(* Logix 5000 AddOnInstructionDefinition export SPEL_Above; software revision 30.01; part 4 of 9 *)

ADD_ON_INSTRUCTION SPEL_Jog   (* revision 1.0, vendor SEIKO EPSON CORP. *)
// Jogs the robot.
VAR_INPUT
   Start : BOOL; {required}
   MaxTime : DINT := 30000; {access None, visible}
END_VAR
VAR_OUTPUT
   InCycle : BOOL; {access Read Only, visible}
   Done : BOOL; {access Read Only, visible}
   Error : BOOL; {access Read Only, visible}
END_VAR
VAR_INPUT
   JogMode : INT; {required}
   Axis : INT; {required}
   Distance : REAL; {required}
END_VAR
VAR_IN_OUT
   ExtInputs : AB:ETHERNET_MODULE_INT_128Bytes:I:0; {required}
   ExtOutputs : AB:ETHERNET_MODULE_INT_128Bytes:O:0; {required}
END_VAR
VAR_OUTPUT
   ErrCode1 : INT; {access Read Only, visible}
   ErrCode2 : INT; {access Read Only, visible}
END_VAR
VAR
   ExecJog : SPEL_ExecCmd := (MaxTime := 3000); {access None}
   Distance_INTS : INT[2]; {access None}
   StartInit : BOOL; {access None}
   OneShotStart : BOOL; {access None}
   Distancex1000 : DINT; {access None}
   ExecTimeout : DINT; {access None}
END_VAR

ROUTINE Logic   (* ladder *)
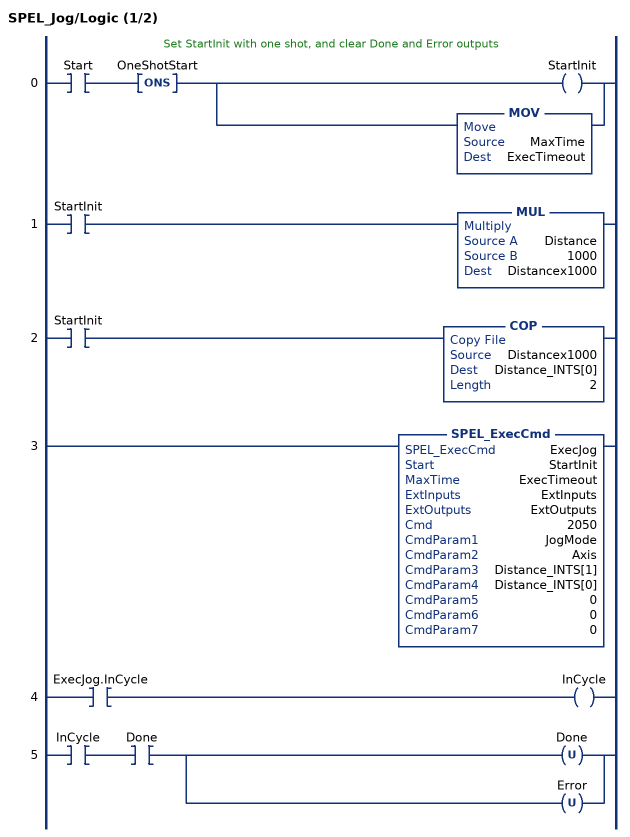
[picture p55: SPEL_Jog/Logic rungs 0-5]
   // Set StartInit with one shot, and clear Done and Error outputs
   0: XIC(Start)ONS(OneShotStart)[OTE(StartInit) ,MOV(MaxTime,ExecTimeout) ];
   1: XIC(StartInit)MUL(Distance,1000,Distancex1000);
   2: XIC(StartInit)COP(Distancex1000,Distance_INTS[0],2);
   3: SPEL_ExecCmd(ExecJog,StartInit,ExecTimeout,ExtInputs,ExtOutputs,2050,JogMode,Axis,Distance_INTS[1],Distance_INTS[0],0,0,0);
   4: XIC(ExecJog.InCycle)OTE(InCycle);
   5: XIC(InCycle)XIC(Done)[OTU(Done) ,OTU(Error) ];
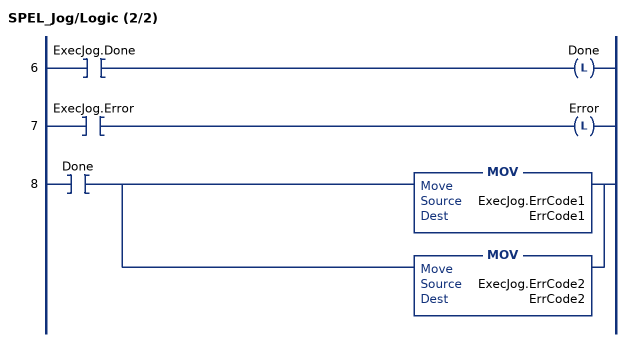
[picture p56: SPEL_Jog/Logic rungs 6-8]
   6: XIC(ExecJog.Done)OTL(Done);
   7: XIC(ExecJog.Error)OTL(Error);
   8: XIC(Done)[MOV(ExecJog.ErrCode1,ErrCode1) ,MOV(ExecJog.ErrCode2,ErrCode2) ];
END_ROUTINE
END_ADD_ON_INSTRUCTION

ADD_ON_INSTRUCTION SPEL_Jump   (* revision 1.0, vendor SEIKO EPSON CORP. *)
// Moves the arm in gate trajectory using PTP motion.
VAR_OUTPUT
   InCycle : BOOL; {access Read Only, visible}
   Done : BOOL; {access Read Only, visible}
   Error : BOOL; {access Read Only, visible}
END_VAR
VAR_INPUT
   Start : BOOL; {required}
   MaxTime : DINT := 30000; {access None, visible}
   TargetType : INT; {access None, visible}
   ArchNum : INT := 7; {access None, visible}
   Point : INT; {required}
   PalletNum : INT; {access None, visible}
   PalletPosOrCol : INT; {access None, visible}
   PalletRow : INT; {access None, visible}
END_VAR
VAR_IN_OUT
   ExtInputs : AB:ETHERNET_MODULE_INT_128Bytes:I:0; {required}
   ExtOutputs : AB:ETHERNET_MODULE_INT_128Bytes:O:0; {required}
END_VAR
VAR_OUTPUT
   ErrCode1 : INT; {access Read Only, visible}
   ErrCode2 : INT; {access Read Only, visible}
END_VAR
VAR
   ExecJump : SPEL_ExecCmd := (MaxTime := 3000, CmdParam1 := 112); {access None}
   StartInit : BOOL; {access None}
   CmdParam1 : INT; {access None}
   PointOrPalletNum : INT; {access None}
   BSL_Control : CONTROL; {access None}
   BSL_SourceBit : BOOL; {access None}
   Local_Arch : DINT; {access None}
   OneShotStart : BOOL; {access None}
   ExecTimeout : DINT; {access None}
   OneShotCP : BOOL; {access None}
   Local_CP : DINT; {access None}
   LocalCP : DINT; {access None}
   ArchError : BOOL; {access None}
   StartExec : BOOL; {access None}
   ExecuteCmd : BOOL; {access None}
   TargetTypeError : BOOL; {access None}
   OneShotArch : BOOL; {access None}
   OneShotTargetType : BOOL; {access None}
END_VAR

ROUTINE Logic   (* ladder *)
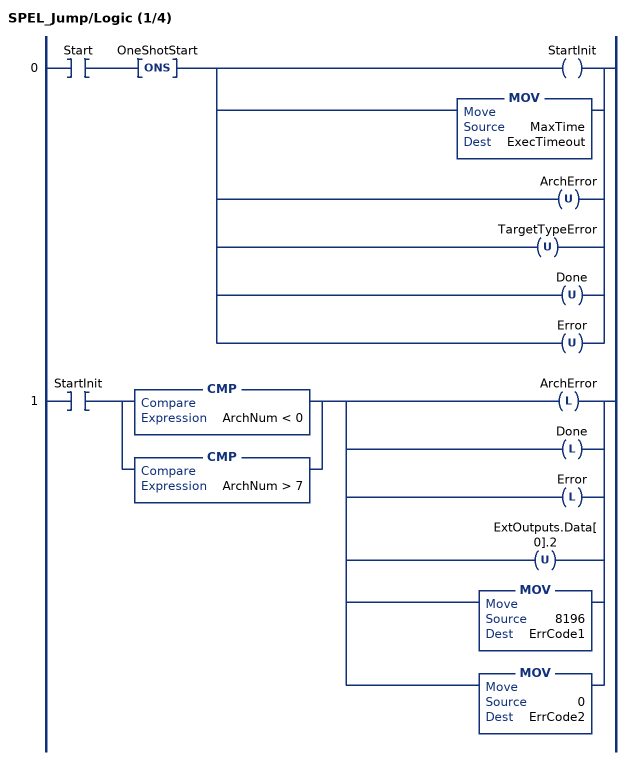
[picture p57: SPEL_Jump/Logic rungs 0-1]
   0: XIC(Start)ONS(OneShotStart)[OTE(StartInit) ,MOV(MaxTime,ExecTimeout) ,OTU(ArchError) ,OTU(TargetTypeError) ,OTU(Done) ,OTU(Error) ];
   1: XIC(StartInit)[CMP(ArchNum < 0) ,CMP(ArchNum > 7) ][OTL(ArchError) ,OTL(Done) ,OTL(Error) ,OTU(ExtOutputs.Data[0].2) ,MOV(8196,ErrCode1) ,MOV(0,ErrCode2) ];
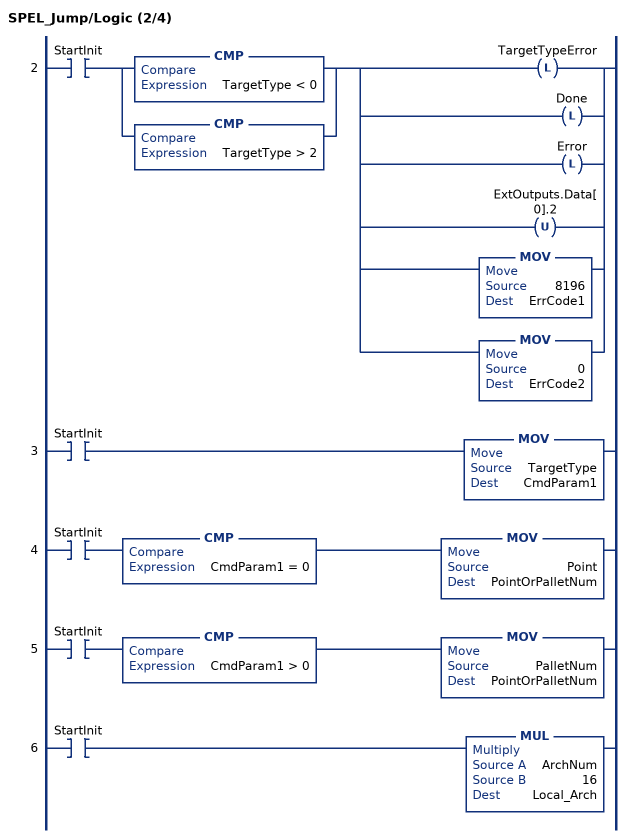
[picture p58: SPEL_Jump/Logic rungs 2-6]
   2: XIC(StartInit)[CMP(TargetType < 0) ,CMP(TargetType > 2) ][OTL(TargetTypeError) ,OTL(Done) ,OTL(Error) ,OTU(ExtOutputs.Data[0].2) ,MOV(8196,ErrCode1) ,MOV(0,ErrCode2) ];
   3: XIC(StartInit)MOV(TargetType,CmdParam1);
   4: XIC(StartInit)CMP(CmdParam1 = 0)MOV(Point,PointOrPalletNum);
   5: XIC(StartInit)CMP(CmdParam1 > 0)MOV(PalletNum,PointOrPalletNum);
   6: XIC(StartInit)MUL(ArchNum,16,Local_Arch);
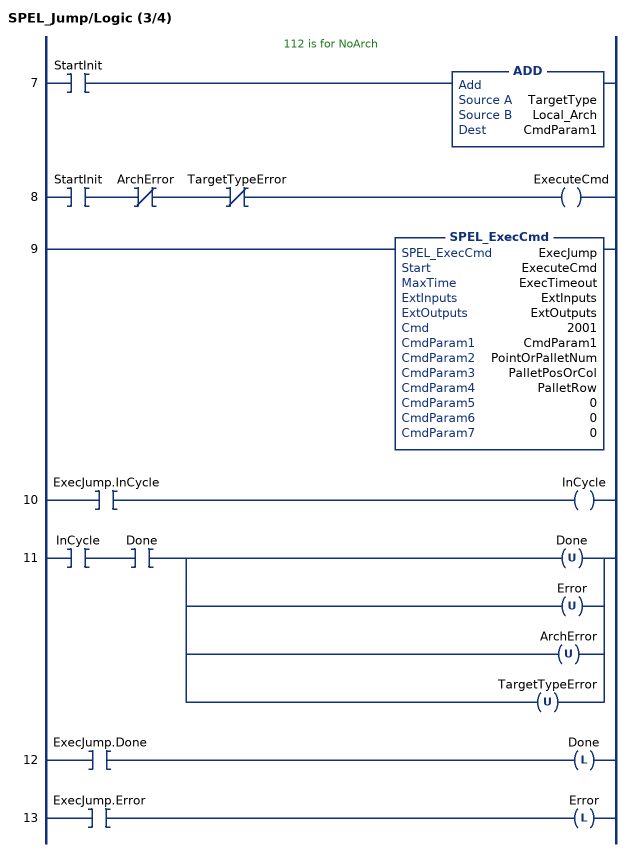
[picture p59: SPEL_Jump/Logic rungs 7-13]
   // 112 is for NoArch
   7: XIC(StartInit)ADD(TargetType,Local_Arch,CmdParam1);
   8: XIC(StartInit)XIO(ArchError)XIO(TargetTypeError)OTE(ExecuteCmd);
   9: SPEL_ExecCmd(ExecJump,ExecuteCmd,ExecTimeout,ExtInputs,ExtOutputs,2001,CmdParam1,PointOrPalletNum,PalletPosOrCol,PalletRow,0,0,0);
   10: XIC(ExecJump.InCycle)OTE(InCycle);
   11: XIC(InCycle)XIC(Done)[OTU(Done) ,OTU(Error) ,OTU(ArchError) ,OTU(TargetTypeError) ];
   12: XIC(ExecJump.Done)OTL(Done);
   13: XIC(ExecJump.Error)OTL(Error);
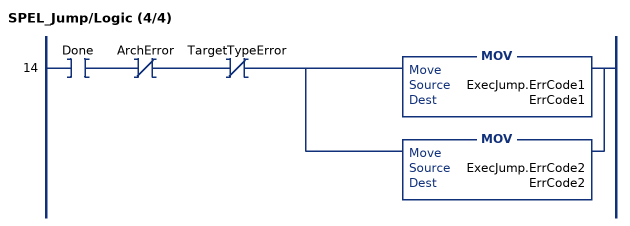
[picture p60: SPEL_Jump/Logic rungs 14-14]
   14: XIC(Done)XIO(ArchError)XIO(TargetTypeError)[MOV(ExecJump.ErrCode1,ErrCode1) ,MOV(ExecJump.ErrCode2,ErrCode2) ];
END_ROUTINE
END_ADD_ON_INSTRUCTION

ADD_ON_INSTRUCTION SPEL_Jump3   (* revision 1.0, vendor SEIKO EPSON CORP. *)
// Moves the arm with 3D gate motion
// This is a combination of two CP motion and one PTP motion.
VAR_OUTPUT
   InCycle : BOOL; {access Read Only, visible}
   Done : BOOL; {access Read Only, visible}
   Error : BOOL; {access Read Only, visible}
END_VAR
VAR_INPUT
   Start : BOOL; {required}
   MaxTime : DINT := 30000; {access None, visible}
   ArchNum : DINT := 7; {access None, visible}
   DepartPoint : INT; {required}
   ApproPoint : INT; {required}
   DestPoint : INT; {required}
END_VAR
VAR_IN_OUT
   ExtInputs : AB:ETHERNET_MODULE_INT_128Bytes:I:0; {required}
   ExtOutputs : AB:ETHERNET_MODULE_INT_128Bytes:O:0; {required}
END_VAR
VAR_OUTPUT
   ErrCode1 : INT; {access Read Only, visible}
   ErrCode2 : INT; {access Read Only, visible}
END_VAR
VAR
   ExecJump3 : SPEL_ExecCmd := (MaxTime := 3000, CmdParam1 := 112); {access None}
   OneShotStart : BOOL; {access None}
   StartInit : BOOL; {access None}
   ExecTimeout : DINT; {access None}
   Local_Arch : DINT; {access None}
   CmdParam1 : DINT; {access None}
   ArchError : BOOL; {access None}
   StartExec : BOOL; {access None}
   ExecuteCmd : BOOL; {access None}
   OneShotArch : BOOL; {access None}
END_VAR

ROUTINE Logic   (* ladder *)
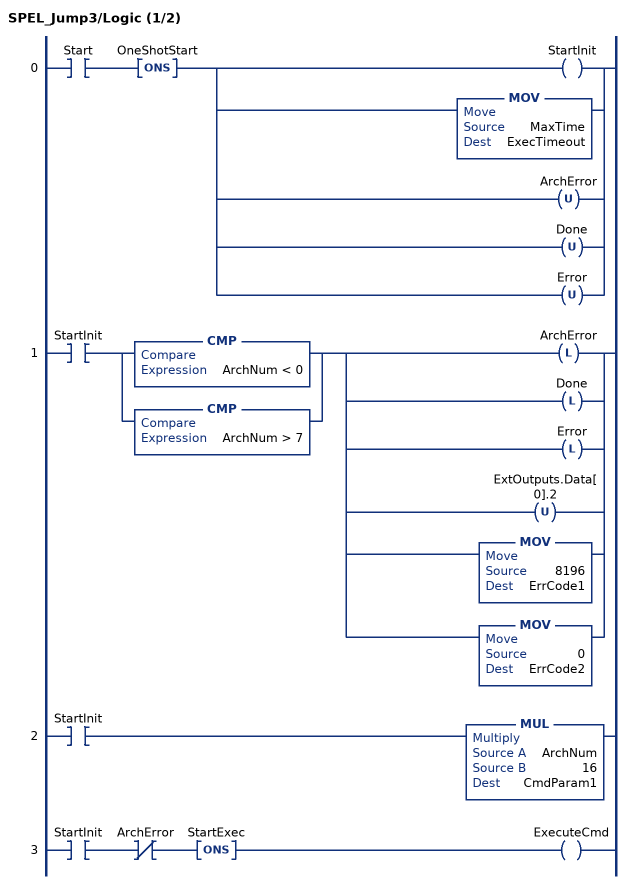
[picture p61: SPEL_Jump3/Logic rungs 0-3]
   0: XIC(Start)ONS(OneShotStart)[OTE(StartInit) ,MOV(MaxTime,ExecTimeout) ,OTU(ArchError) ,OTU(Done) ,OTU(Error) ];
   1: XIC(StartInit)[CMP(ArchNum < 0) ,CMP(ArchNum > 7) ][OTL(ArchError) ,OTL(Done) ,OTL(Error) ,OTU(ExtOutputs.Data[0].2) ,MOV(8196,ErrCode1) ,MOV(0,ErrCode2) ];
   2: XIC(StartInit)MUL(ArchNum,16,CmdParam1);
   3: XIC(StartInit)XIO(ArchError)ONS(StartExec)OTE(ExecuteCmd);
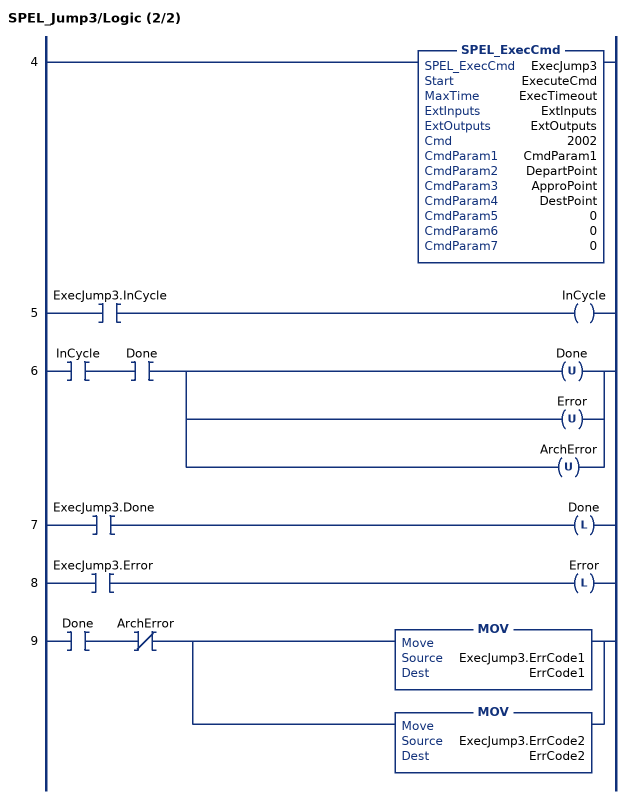
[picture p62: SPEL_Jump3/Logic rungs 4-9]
   4: SPEL_ExecCmd(ExecJump3,ExecuteCmd,ExecTimeout,ExtInputs,ExtOutputs,2002,CmdParam1,DepartPoint,ApproPoint,DestPoint,0,0,0);
   5: XIC(ExecJump3.InCycle)OTE(InCycle);
   6: XIC(InCycle)XIC(Done)[OTU(Done) ,OTU(Error) ,OTU(ArchError) ];
   7: XIC(ExecJump3.Done)OTL(Done);
   8: XIC(ExecJump3.Error)OTL(Error);
   9: XIC(Done)XIO(ArchError)[MOV(ExecJump3.ErrCode1,ErrCode1) ,MOV(ExecJump3.ErrCode2,ErrCode2) ];
END_ROUTINE
END_ADD_ON_INSTRUCTION

ADD_ON_INSTRUCTION SPEL_Jump3CP   (* revision 1.0, vendor SEIKO EPSON CORP. *)
// Moves the manipulator in 3D gate trajectory, using three CP motions.
VAR_OUTPUT
   InCycle : BOOL; {access Read Only, visible}
   Done : BOOL; {access Read Only, visible}
   Error : BOOL; {access Read Only, visible}
END_VAR
VAR_INPUT
   Start : BOOL; {required}
   MaxTime : DINT := 120000; {access None, visible}
   ArchNum : DINT := 7; {access None, visible}
   DepartPoint : INT; {required}
   ApproPoint : INT; {required}
   DestPoint : INT; {required}
END_VAR
VAR_IN_OUT
   ExtInputs : AB:ETHERNET_MODULE_INT_128Bytes:I:0; {required}   // ExtReset Bit
   ExtOutputs : AB:ETHERNET_MODULE_INT_128Bytes:O:0; {required}
END_VAR
VAR_OUTPUT
   ErrCode1 : INT; {access Read Only, visible}
   ErrCode2 : INT; {access Read Only, visible}
END_VAR
VAR
   ExecJump3CP : SPEL_ExecCmd := (MaxTime := 3000, CmdParam1 := 112); {access None}
   OneShotStart : BOOL; {access None}
   StartInit : BOOL; {access None}
   ExecTimeout : DINT; {access None}
   Local_Arch : DINT; {access None}
   CmdParam1 : DINT; {access None}
   StartExec : BOOL; {access None}
   ExecuteCmd : BOOL; {access None}
   ArchError : BOOL; {access None}
   OneShotArch : BOOL; {access None}
END_VAR

ROUTINE Logic   (* ladder *)
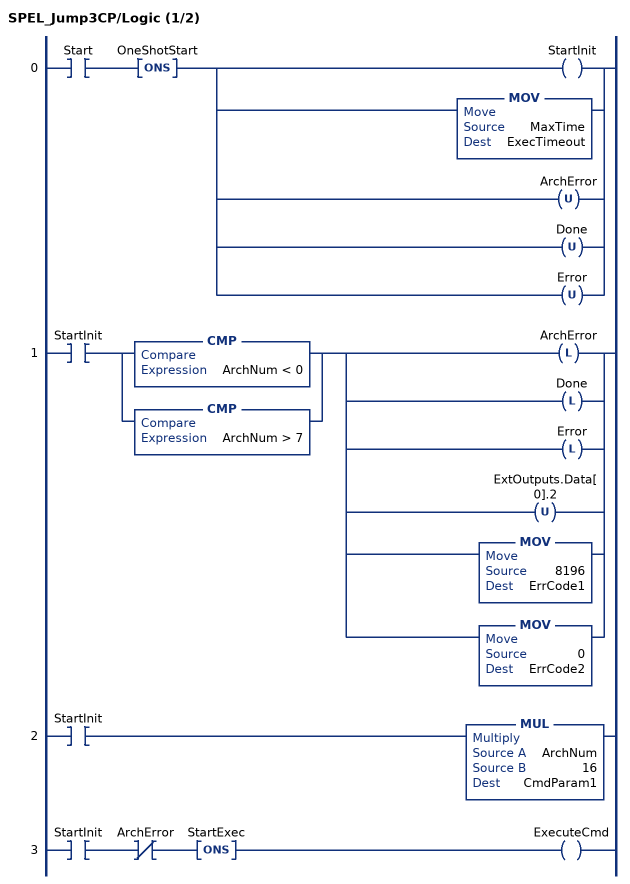
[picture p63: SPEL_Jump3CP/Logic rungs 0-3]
   0: XIC(Start)ONS(OneShotStart)[OTE(StartInit) ,MOV(MaxTime,ExecTimeout) ,OTU(ArchError) ,OTU(Done) ,OTU(Error) ];
   1: XIC(StartInit)[CMP(ArchNum < 0) ,CMP(ArchNum > 7) ][OTL(ArchError) ,OTL(Done) ,OTL(Error) ,OTU(ExtOutputs.Data[0].2) ,MOV(8196,ErrCode1) ,MOV(0,ErrCode2) ];
   2: XIC(StartInit)MUL(ArchNum,16,CmdParam1);
   3: XIC(StartInit)XIO(ArchError)ONS(StartExec)OTE(ExecuteCmd);
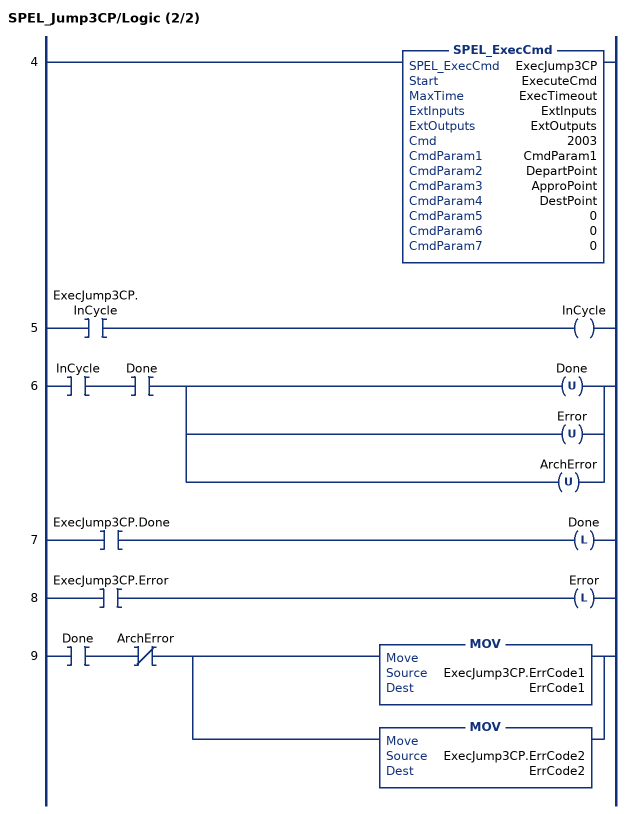
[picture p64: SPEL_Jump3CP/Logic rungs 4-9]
   4: SPEL_ExecCmd(ExecJump3CP,ExecuteCmd,ExecTimeout,ExtInputs,ExtOutputs,2003,CmdParam1,DepartPoint,ApproPoint,DestPoint,0,0,0);
   5: XIC(ExecJump3CP.InCycle)OTE(InCycle);
   6: XIC(InCycle)XIC(Done)[OTU(Done) ,OTU(Error) ,OTU(ArchError) ];
   7: XIC(ExecJump3CP.Done)OTL(Done);
   8: XIC(ExecJump3CP.Error)OTL(Error);
   9: XIC(Done)XIO(ArchError)[MOV(ExecJump3CP.ErrCode1,ErrCode1) ,MOV(ExecJump3CP.ErrCode2,ErrCode2) ];
END_ROUTINE
END_ADD_ON_INSTRUCTION

ADD_ON_INSTRUCTION SPEL_Lefty   (* revision 1.0, vendor SEIKO EPSON CORP. *)
// Sets the hand orientation of the specified point to Lefty.
VAR_OUTPUT
   InCycle : BOOL; {access Read Only, visible}
   Done : BOOL; {access Read Only, visible}
   Error : BOOL; {access Read Only, visible}
END_VAR
VAR_INPUT
   Start : BOOL; {required}
   Point : INT; {required}
END_VAR
VAR_IN_OUT
   ExtInputs : AB:ETHERNET_MODULE_INT_128Bytes:I:0; {required}
   ExtOutputs : AB:ETHERNET_MODULE_INT_128Bytes:O:0; {required}
END_VAR
VAR_OUTPUT
   ErrCode1 : INT; {access Read Only, visible}
   ErrCode2 : INT; {access Read Only, visible}
END_VAR
VAR
   ExecLefty : SPEL_ExecCmd := (MaxTime := 3000); {access None}
   height_INTS : INT[2]; {access None}
   OneShotStart : BOOL; {access None}
   StartCoil : BOOL; {access None}
   ExecTimeout : DINT; {access None}
END_VAR

ROUTINE Logic   (* ladder *)
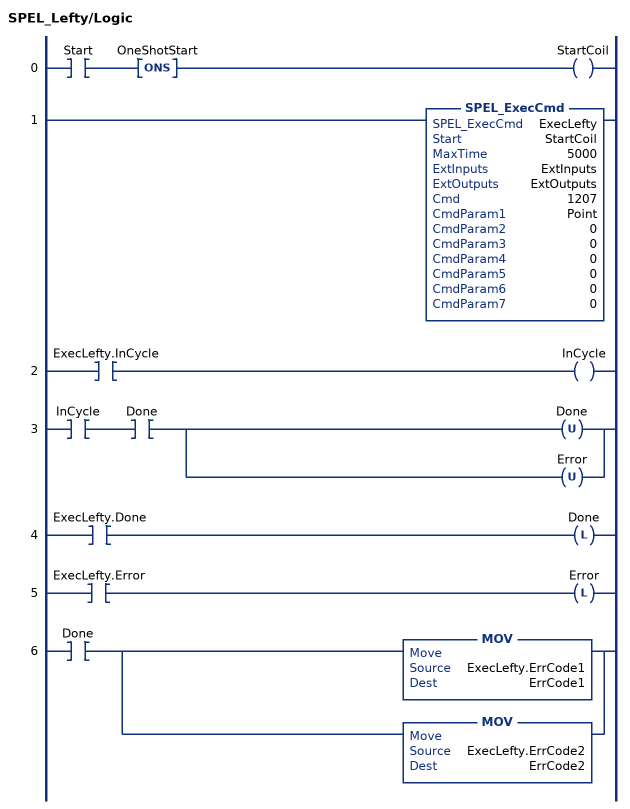
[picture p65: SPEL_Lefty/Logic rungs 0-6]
   0: XIC(Start)ONS(OneShotStart)OTE(StartCoil);
   1: SPEL_ExecCmd(ExecLefty,StartCoil,5000,ExtInputs,ExtOutputs,1207,Point,0,0,0,0,0,0);
   2: XIC(ExecLefty.InCycle)OTE(InCycle);
   3: XIC(InCycle)XIC(Done)[OTU(Done) ,OTU(Error) ];
   4: XIC(ExecLefty.Done)OTL(Done);
   5: XIC(ExecLefty.Error)OTL(Error);
   6: XIC(Done)[MOV(ExecLefty.ErrCode1,ErrCode1) ,MOV(ExecLefty.ErrCode2,ErrCode2) ];
END_ROUTINE
END_ADD_ON_INSTRUCTION

ADD_ON_INSTRUCTION SPEL_LimZ   (* revision 1.0, vendor SEIKO EPSON CORP. *)
// Sets the initial Joint #3 height (Z coordinate value) in Jump command.
VAR_OUTPUT
   InCycle : BOOL; {access Read Only, visible}
   Done : BOOL; {access Read Only, visible}
   Error : BOOL; {access Read Only, visible}
END_VAR
VAR_INPUT
   Start : BOOL; {required}
   Height : REAL; {required}
END_VAR
VAR_IN_OUT
   ExtInputs : AB:ETHERNET_MODULE_INT_128Bytes:I:0; {required}
   ExtOutputs : AB:ETHERNET_MODULE_INT_128Bytes:O:0; {required}
END_VAR
VAR_OUTPUT
   ErrCode1 : INT; {access Read Only, visible}
   ErrCode2 : INT; {access Read Only, visible}
END_VAR
VAR
   ExecLimZ : SPEL_ExecCmd := (MaxTime := 3000); {access None}
   StartInit : BOOL; {access None}
   OneShotStart : BOOL; {access None}
   heightx1000 : DINT; {access None}
   height_INTS : INT[2]; {access None}
   ExecTimeout : DINT; {access None}
END_VAR

ROUTINE Logic   (* ladder *)
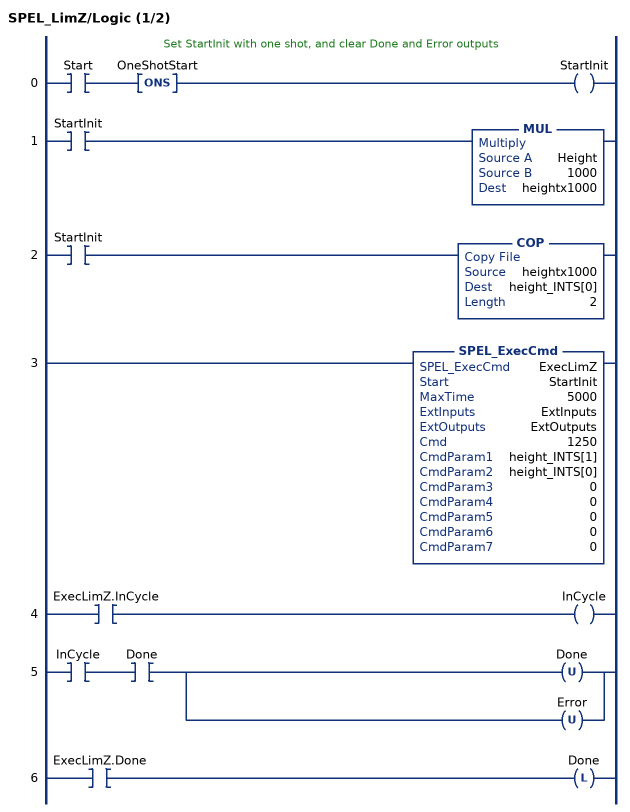
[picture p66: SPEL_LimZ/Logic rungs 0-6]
   // Set StartInit with one shot, and clear Done and Error outputs
   0: XIC(Start)ONS(OneShotStart)OTE(StartInit);
   1: XIC(StartInit)MUL(Height,1000,heightx1000);
   2: XIC(StartInit)COP(heightx1000,height_INTS[0],2);
   3: SPEL_ExecCmd(ExecLimZ,StartInit,5000,ExtInputs,ExtOutputs,1250,height_INTS[1],height_INTS[0],0,0,0,0,0);
   4: XIC(ExecLimZ.InCycle)OTE(InCycle);
   5: XIC(InCycle)XIC(Done)[OTU(Done) ,OTU(Error) ];
   6: XIC(ExecLimZ.Done)OTL(Done);
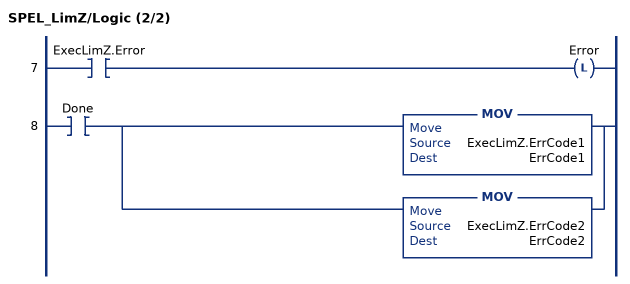
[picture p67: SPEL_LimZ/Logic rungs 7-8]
   7: XIC(ExecLimZ.Error)OTL(Error);
   8: XIC(Done)[MOV(ExecLimZ.ErrCode1,ErrCode1) ,MOV(ExecLimZ.ErrCode2,ErrCode2) ];
END_ROUTINE
END_ADD_ON_INSTRUCTION

ADD_ON_INSTRUCTION SPEL_LocalGet   (* revision 1.0, vendor SEIKO EPSON CORP. *)
// Gets the setting status of the Local coordinate system number.
VAR_INPUT
   Start : BOOL; {required}
END_VAR
VAR_OUTPUT
   InCycle : BOOL; {access Read Only, visible}
   Done : BOOL; {access Read Only, visible}
   Error : BOOL; {access Read Only, visible}
END_VAR
VAR_INPUT
   NumAxes : INT; {required}
   LocalNum : INT; {required}
END_VAR
VAR_OUTPUT
   LocalX : REAL; {visible}
   LocalY : REAL; {visible}
   LocalZ : REAL; {visible}
   LocalU : REAL; {visible}
   LocalV : REAL; {visible}
   LocalW : REAL; {visible}
END_VAR
VAR_IN_OUT
   ExtInputs : AB:ETHERNET_MODULE_INT_128Bytes:I:0; {required}
   ExtOutputs : AB:ETHERNET_MODULE_INT_128Bytes:O:0; {required}
END_VAR
VAR_OUTPUT
   ErrCode1 : INT; {access Read Only, visible}
   ErrCode2 : INT; {access Read Only, visible}
END_VAR
VAR
   Coordinatex1000 : DINT; {access None}
   Coordinate_INTS : INT[2]; {access None}
   ExecLocalGetZ : SPEL_ExecCmd := (MaxTime := 3000); {access None}
   ExecLocalGetY : SPEL_ExecCmd := (MaxTime := 3000); {access None}
   ExecLocalGetX : SPEL_ExecCmd := (MaxTime := 3000); {access None}
   X6 : BOOL; {access None}
   StartInit : BOOL[32]; {access None}
   OneShotStart : BOOL[32]; {access None}
   ExecLocalGetW : SPEL_ExecCmd := (MaxTime := 3000); {access None}
   ExecLocalGetV : SPEL_ExecCmd := (MaxTime := 3000); {access None}
   ExecLocalGetU : SPEL_ExecCmd := (MaxTime := 3000); {access None}
   ExecTimeout : DINT; {access None}
END_VAR

ROUTINE Logic   (* ladder *)
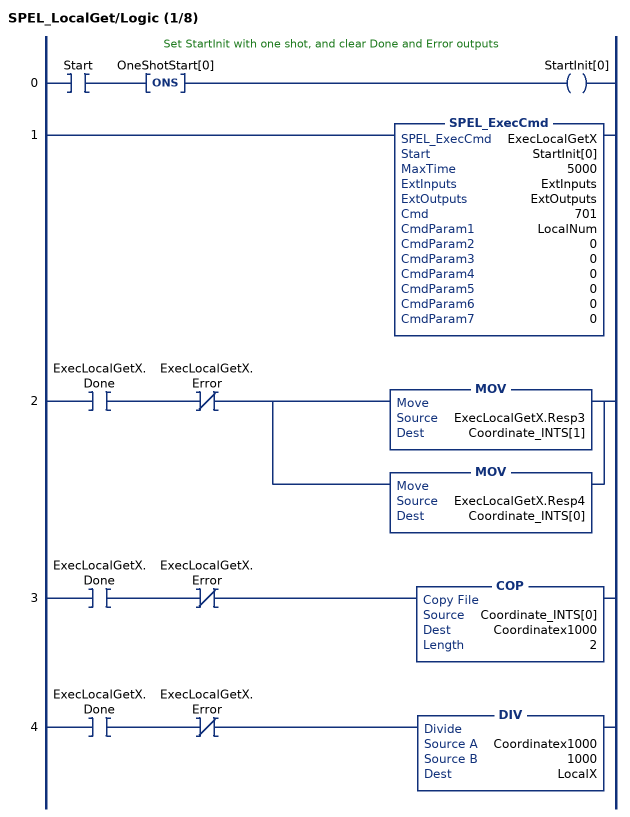
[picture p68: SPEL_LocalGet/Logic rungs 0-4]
   // Set StartInit with one shot, and clear Done and Error outputs
   0: XIC(Start)ONS(OneShotStart[0])OTE(StartInit[0]);
   1: SPEL_ExecCmd(ExecLocalGetX,StartInit[0],5000,ExtInputs,ExtOutputs,701,LocalNum,0,0,0,0,0,0);
   2: XIC(ExecLocalGetX.Done)XIO(ExecLocalGetX.Error)[MOV(ExecLocalGetX.Resp3,Coordinate_INTS[1]) ,MOV(ExecLocalGetX.Resp4,Coordinate_INTS[0]) ];
   3: XIC(ExecLocalGetX.Done)XIO(ExecLocalGetX.Error)COP(Coordinate_INTS[0],Coordinatex1000,2);
   4: XIC(ExecLocalGetX.Done)XIO(ExecLocalGetX.Error)DIV(Coordinatex1000,1000,LocalX);
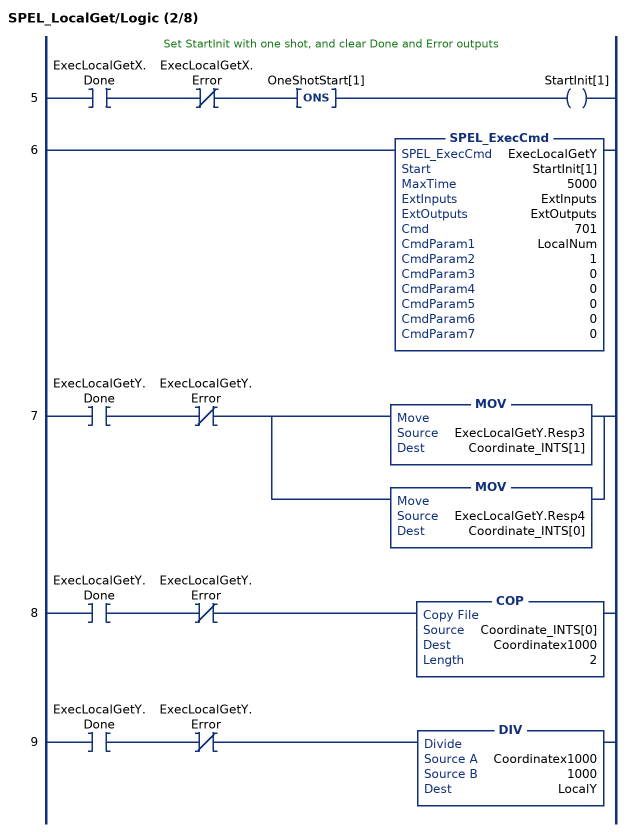
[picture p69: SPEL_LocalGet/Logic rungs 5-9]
   // Set StartInit with one shot, and clear Done and Error outputs
   5: XIC(ExecLocalGetX.Done)XIO(ExecLocalGetX.Error)ONS(OneShotStart[1])OTE(StartInit[1]);
   6: SPEL_ExecCmd(ExecLocalGetY,StartInit[1],5000,ExtInputs,ExtOutputs,701,LocalNum,1,0,0,0,0,0);
   7: XIC(ExecLocalGetY.Done)XIO(ExecLocalGetY.Error)[MOV(ExecLocalGetY.Resp3,Coordinate_INTS[1]) ,MOV(ExecLocalGetY.Resp4,Coordinate_INTS[0]) ];
   8: XIC(ExecLocalGetY.Done)XIO(ExecLocalGetY.Error)COP(Coordinate_INTS[0],Coordinatex1000,2);
   9: XIC(ExecLocalGetY.Done)XIO(ExecLocalGetY.Error)DIV(Coordinatex1000,1000,LocalY);
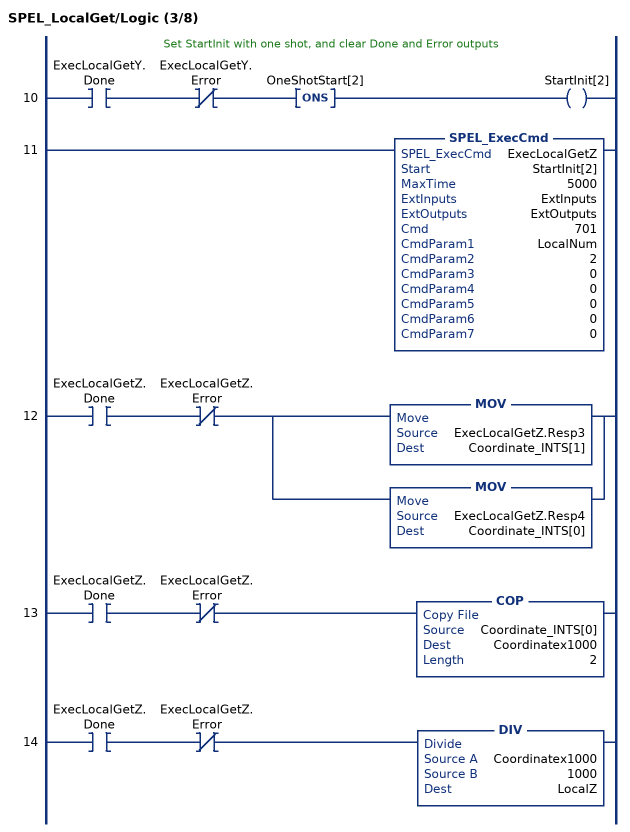
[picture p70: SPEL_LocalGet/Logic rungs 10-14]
   // Set StartInit with one shot, and clear Done and Error outputs
   10: XIC(ExecLocalGetY.Done)XIO(ExecLocalGetY.Error)ONS(OneShotStart[2])OTE(StartInit[2]);
   11: SPEL_ExecCmd(ExecLocalGetZ,StartInit[2],5000,ExtInputs,ExtOutputs,701,LocalNum,2,0,0,0,0,0);
   12: XIC(ExecLocalGetZ.Done)XIO(ExecLocalGetZ.Error)[MOV(ExecLocalGetZ.Resp3,Coordinate_INTS[1]) ,MOV(ExecLocalGetZ.Resp4,Coordinate_INTS[0]) ];
   13: XIC(ExecLocalGetZ.Done)XIO(ExecLocalGetZ.Error)COP(Coordinate_INTS[0],Coordinatex1000,2);
   14: XIC(ExecLocalGetZ.Done)XIO(ExecLocalGetZ.Error)DIV(Coordinatex1000,1000,LocalZ);
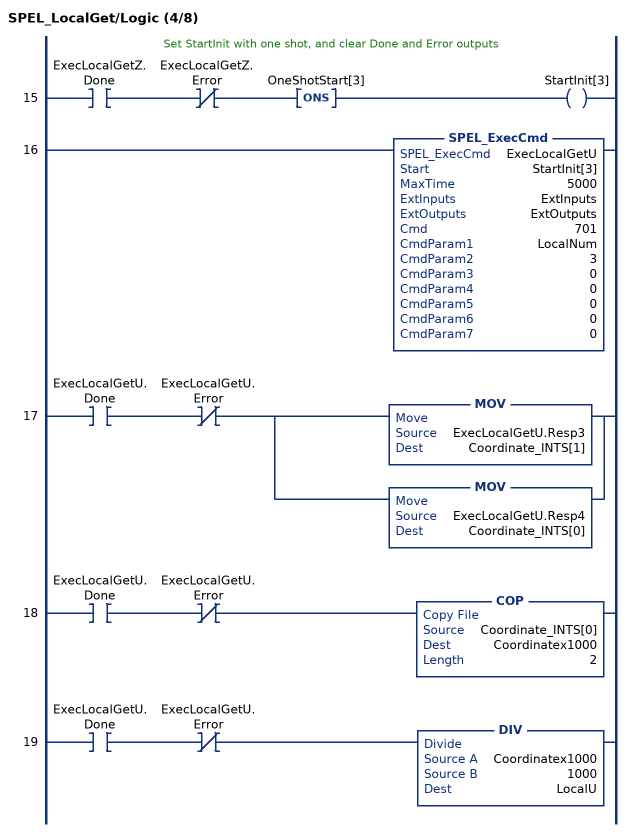
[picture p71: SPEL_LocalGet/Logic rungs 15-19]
   // Set StartInit with one shot, and clear Done and Error outputs
   15: XIC(ExecLocalGetZ.Done)XIO(ExecLocalGetZ.Error)ONS(OneShotStart[3])OTE(StartInit[3]);
   16: SPEL_ExecCmd(ExecLocalGetU,StartInit[3],5000,ExtInputs,ExtOutputs,701,LocalNum,3,0,0,0,0,0);
   17: XIC(ExecLocalGetU.Done)XIO(ExecLocalGetU.Error)[MOV(ExecLocalGetU.Resp3,Coordinate_INTS[1]) ,MOV(ExecLocalGetU.Resp4,Coordinate_INTS[0]) ];
   18: XIC(ExecLocalGetU.Done)XIO(ExecLocalGetU.Error)COP(Coordinate_INTS[0],Coordinatex1000,2);
   19: XIC(ExecLocalGetU.Done)XIO(ExecLocalGetU.Error)DIV(Coordinatex1000,1000,LocalU);
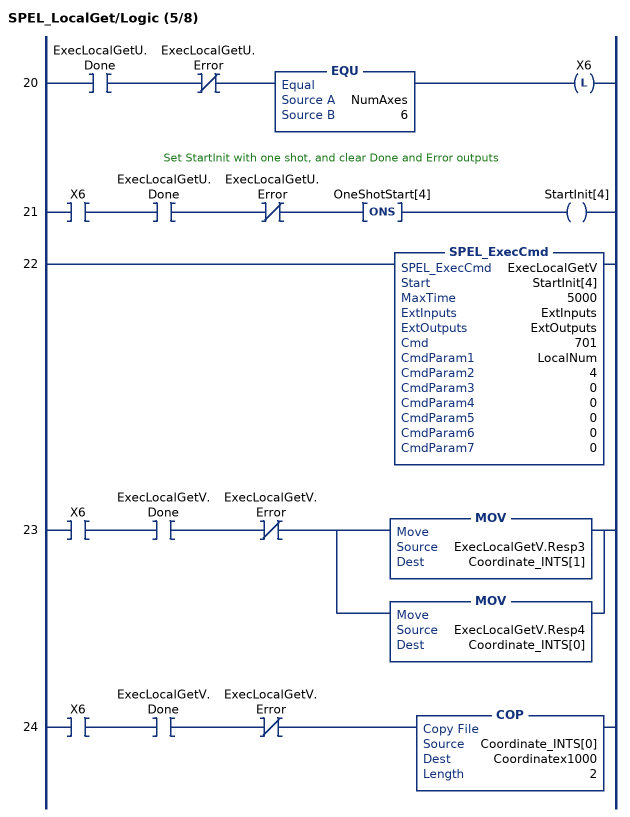
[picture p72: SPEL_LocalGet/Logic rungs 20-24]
   20: XIC(ExecLocalGetU.Done)XIO(ExecLocalGetU.Error)EQU(NumAxes,6)OTL(X6);
   // Set StartInit with one shot, and clear Done and Error outputs
   21: XIC(X6)XIC(ExecLocalGetU.Done)XIO(ExecLocalGetU.Error)ONS(OneShotStart[4])OTE(StartInit[4]);
   22: SPEL_ExecCmd(ExecLocalGetV,StartInit[4],5000,ExtInputs,ExtOutputs,701,LocalNum,4,0,0,0,0,0);
   23: XIC(X6)XIC(ExecLocalGetV.Done)XIO(ExecLocalGetV.Error)[MOV(ExecLocalGetV.Resp3,Coordinate_INTS[1]) ,MOV(ExecLocalGetV.Resp4,Coordinate_INTS[0]) ];
   24: XIC(X6)XIC(ExecLocalGetV.Done)XIO(ExecLocalGetV.Error)COP(Coordinate_INTS[0],Coordinatex1000,2);
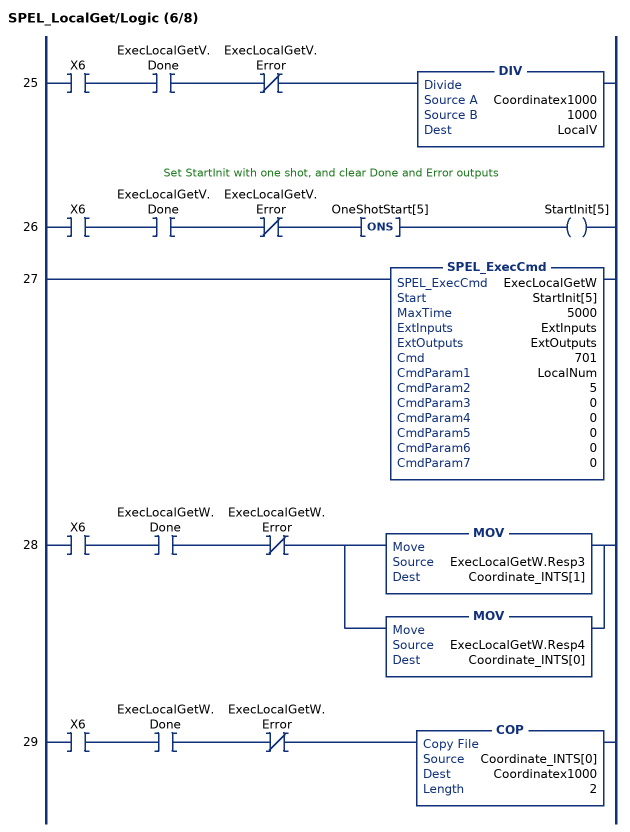
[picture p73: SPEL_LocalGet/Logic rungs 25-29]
   25: XIC(X6)XIC(ExecLocalGetV.Done)XIO(ExecLocalGetV.Error)DIV(Coordinatex1000,1000,LocalV);
   // Set StartInit with one shot, and clear Done and Error outputs
   26: XIC(X6)XIC(ExecLocalGetV.Done)XIO(ExecLocalGetV.Error)ONS(OneShotStart[5])OTE(StartInit[5]);
   27: SPEL_ExecCmd(ExecLocalGetW,StartInit[5],5000,ExtInputs,ExtOutputs,701,LocalNum,5,0,0,0,0,0);
   28: XIC(X6)XIC(ExecLocalGetW.Done)XIO(ExecLocalGetW.Error)[MOV(ExecLocalGetW.Resp3,Coordinate_INTS[1]) ,MOV(ExecLocalGetW.Resp4,Coordinate_INTS[0]) ];
   29: XIC(X6)XIC(ExecLocalGetW.Done)XIO(ExecLocalGetW.Error)COP(Coordinate_INTS[0],Coordinatex1000,2);
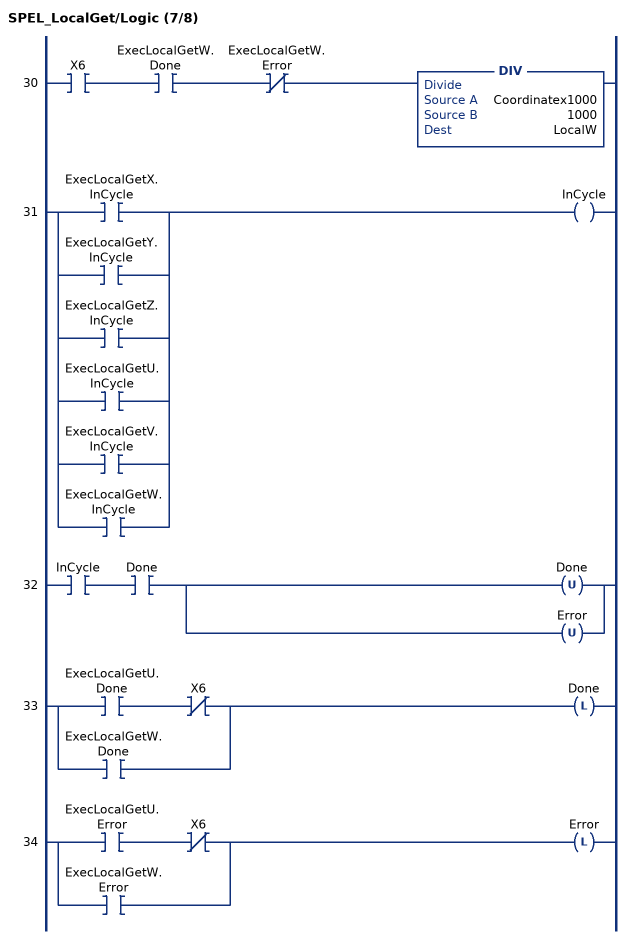
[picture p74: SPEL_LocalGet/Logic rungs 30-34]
   30: XIC(X6)XIC(ExecLocalGetW.Done)XIO(ExecLocalGetW.Error)DIV(Coordinatex1000,1000,LocalW);
   31: [XIC(ExecLocalGetX.InCycle) ,XIC(ExecLocalGetY.InCycle) ,XIC(ExecLocalGetZ.InCycle) ,XIC(ExecLocalGetU.InCycle) ,XIC(ExecLocalGetV.InCycle) ,XIC(ExecLocalGetW.InCycle) ]OTE(InCycle);
   32: XIC(InCycle)XIC(Done)[OTU(Done) ,OTU(Error) ];
   33: [XIC(ExecLocalGetU.Done) XIO(X6) ,XIC(ExecLocalGetW.Done) ]OTL(Done);
   34: [XIC(ExecLocalGetU.Error) XIO(X6) ,XIC(ExecLocalGetW.Error) ]OTL(Error);
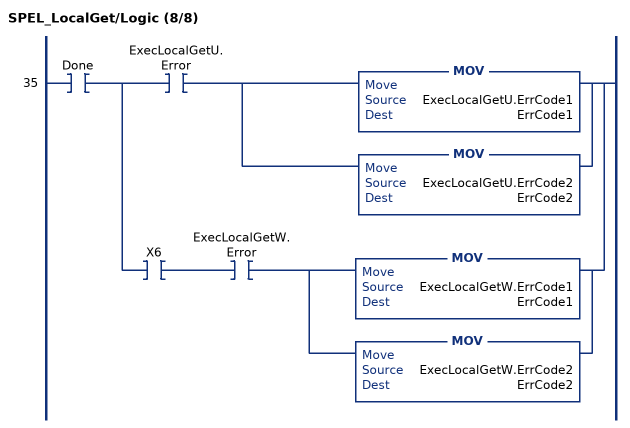
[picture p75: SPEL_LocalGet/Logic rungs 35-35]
   35: XIC(Done)[XIC(ExecLocalGetU.Error) [MOV(ExecLocalGetU.ErrCode1,ErrCode1) ,MOV(ExecLocalGetU.ErrCode2,ErrCode2) ] ,XIC(X6) XIC(ExecLocalGetW.Error) [MOV(ExecLocalGetW.ErrCode1,ErrCode1) ,MOV(ExecLocalGetW.ErrCode2,ErrCode2) ] ];
END_ROUTINE
END_ADD_ON_INSTRUCTION
